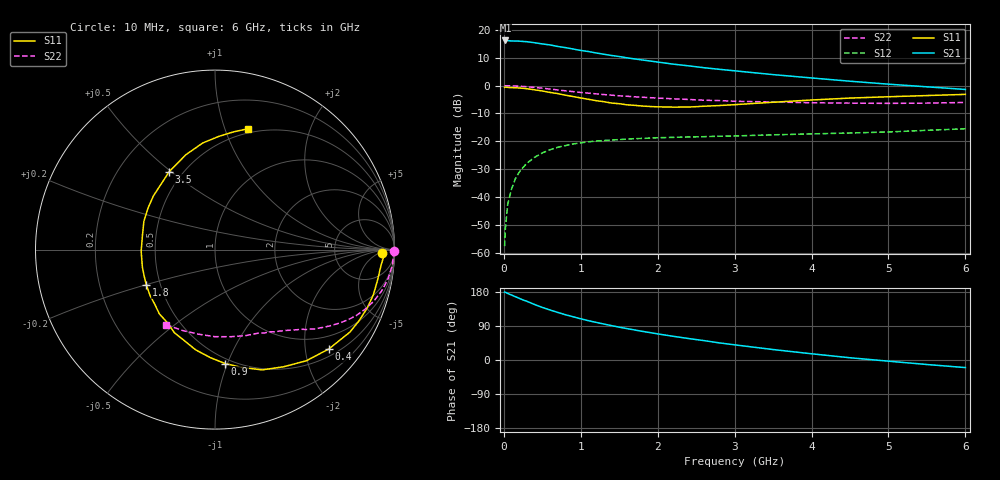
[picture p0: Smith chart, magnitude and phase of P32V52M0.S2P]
! SIEMENS Small Signal Semiconductors
! BFP181
! Si NPN RF Bipolar Junction Transistor in SOT143
! VCE = 2.5 V  IC = 2 mA
! Common Emitter S-Parameters:  March  1996
# GHz  S  MA  R  50
!  f  S11  S21  S12  S22
! GHz  MAG  ANG  MAG  ANG  MAG  ANG  MAG  ANG
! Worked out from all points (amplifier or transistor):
!   36 points, 10 MHz to 6 GHz, reference 50 ohm
!   highest |S21| = 16.3 dB at 20 MHz (marker M1)
!   |S21| within 3 dB of that: start of sweep to 885.2 MHz
!   unconditionally stable (mu >= 1): 2.438 GHz to end of sweep
!   at 250 MHz: K = 0.12, MSG = 22.6 dB, |S12| = -29.4 dB
!   at 1.4 GHz: K = 0.65, MSG = 15.2 dB, |S12| = -19.5 dB
!   at 6 GHz: K = 1.14, MAG = 4.8 dB, |S12| = -15.5 dB
!   lowest NFmin = 1.35 dB at 450 MHz
!   S11 on the Smith chart (normalised r, x): 10 MHz: 25, -8; 400 MHz: 0.66, -2.52; 900 MHz: 0.46, -0.98; 1.8 GHz: 0.42, -0.20; 3.5 GHz: 0.42, +0.49; 6 GHz: 0.46, +1.20
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0.01  0.9307 -1.3  6.454 179.3  0.0013 78.4  0.9966 -0.4
0.02  0.9426 -2.0  6.498 178.8  0.0027 85.6  0.9939 -1.0
0.05  0.9298 -5.2  6.442 175.6  0.0073 89.1  0.9939 -2.4
0.15  0.9176 -15.9  6.339 167.0  0.0212 79.8  0.9848 -7.2
0.2  0.9081 -21.1  6.317 162.8  0.0279 77.3  0.9782 -9.4
0.25  0.8953 -26.3  6.236 158.4  0.0339 74.5  0.9673 -11.7
0.3  0.8809 -31.5  6.173 154.9  0.0404 71.1  0.9568 -13.9
0.4  0.8419 -41.1  5.915 146.4  0.0516 65.9  0.9302 -18.0
0.5  0.8016 -50.6  5.63 138.8  0.0617 59.9  0.9003 -21.6
0.6  0.7562 -59.7  5.401 132.0  0.0705 55.3  0.8689 -25.0
0.8  0.674 -77.0  4.833 119.5  0.0837 47.2  0.8084 -30.3
0.9  0.6376 -84.9  4.561 114.1  0.0895 43.9  0.7813 -32.5
1.1  0.5686 -101.0  4.108 103.7  0.0979 38.3  0.7335 -36.4
1.4  0.4863 -123.0  3.491 90.7  0.1055 31.8  0.6745 -41.3
1.6  0.4527 -138.0  3.168 82.9  0.1095 28.9  0.645 -43.7
1.8  0.4304 -152.6  2.895 75.6  0.1126 26.5  0.6193 -46.3
2.2  0.4114 -178.7  2.44 62.6  0.1176 22.6  0.58 -51.5
2.8  0.4389 148.3  1.969 45.2  0.1232 18.8  0.5388 -59.7
3.5  0.5034 120.5  1.58 27.6  0.1306 16.2  0.5084 -70.6
4.5  0.5983 96.5  1.202 5.9  0.1409 12.8  0.485 -90.3
5.5  0.6638 81.1  0.953 -11.9  0.1574 11.5  0.4855 -111.7
6  0.6971 74.9  0.855 -20.0  0.1679 9.4  0.4989 -122.9
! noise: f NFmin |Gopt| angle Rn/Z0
0.45  1.35  0.6  17  0.4
0.9  1.45  0.5  36  0.4
1.8  1.8  0.31  80  0.37
